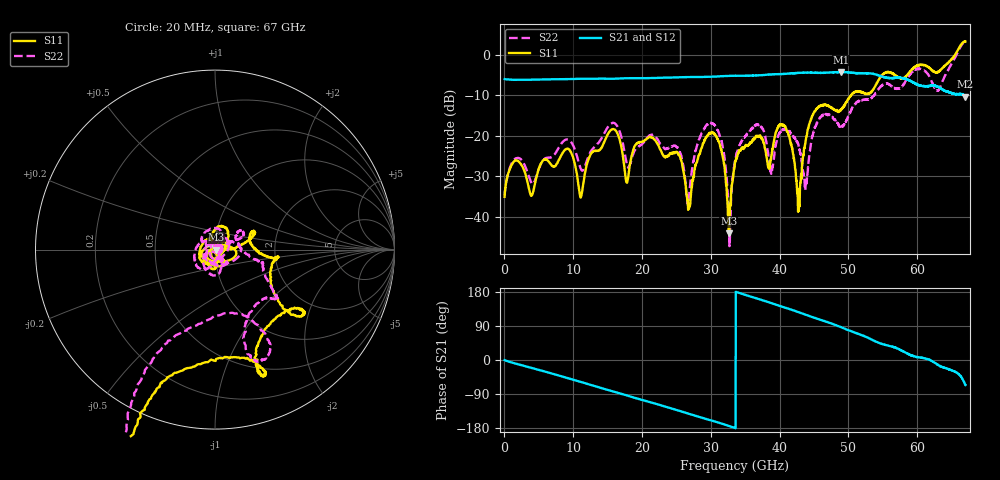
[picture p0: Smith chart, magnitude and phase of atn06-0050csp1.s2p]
!Keysight Technologies,N5247B,US58420632,A.14.00.23
!Date: Monday, April 25, 2022 11:31:55
!Correction: S11(C  2-Port  )
!S21(C  2-Port  )
!S12(C  2-Port  )
!S22(C  2-Port  )
!S2P File: Measurement: :
# Hz S  dB  R 50
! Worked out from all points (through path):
!   3350 points, 20 MHz to 67 GHz, reference 50 ohm
!   highest |S21| = -4.23 dB at 48.9 GHz (marker M1); lowest = -10.4 dB at 67 GHz (marker M2)
!   group delay of S21, straight-line fit = 16.5 ps
!   lowest |S11| = -44.1 dB at 32.6 GHz (marker M3), VSWR 1.01, Z = 50.6 - j0.0115 ohm
!   |S11| at or under -10 dB: start of sweep to 50.39 GHz
!   |S22| runs from -47.3 to 3.6 dB; largest |S21 - S12| = 0.0066
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2e7  -35.09 7.4  -5.99 -0.3  -5.99 -0.3  -34.72 6.2
9.1e9  -23.19 27.8  -6.00 -47.3  -6.00 -47.3  -20.91 36.7
1.12e10  -34.67 147.7  -5.90 -58.4  -5.91 -58.4  -28.47 130.2
1.554e10  -18.47 -17.6  -5.91 -81.6  -5.92 -81.6  -16.96 -9.7
1.778e10  -31.57 98.0  -5.78 -93.4  -5.78 -93.4  -26.99 84.1
2.236e10  -22.23 -50.6  -5.69 -117.5  -5.69 -117.5  -21.17 -44.9
2.536e10  -24.66 -67.1  -5.56 -133.8  -5.56 -133.8  -23.57 -49.9
2.668e10  -38.09 -101.3  -5.49 -141.2  -5.50 -141.2  -36.84 -109.2
3.042e10  -19.39 -89.9  -5.39 -161.4  -5.40 -161.4  -17.23 -83.7
3.178e10  -25.71 -78.5  -5.25 -169.0  -5.27 -169.1  -23.31 -61.6
3.26e10  -44.06 -1.0  -5.21 -173.8  -5.21 -173.9  -39.57 -18.0
3.352e10  -26.37 97.3  -5.18 -179.6  -5.17 -179.5  -26.20 129.7
3.688e10  -20.03 -138.1  -5.09 161.3  -5.07 161.4  -17.33 -132.4
3.88e10  -24.94 12.4  -4.86 149.8  -4.84 149.8  -29.19 -19.3
4.052e10  -17.30 73.5  -4.72 139.6  -4.73 139.6  -18.42 86.7
4.276e10  -38.41 55.7  -4.48 126.3  -4.45 126.3  -22.65 153.4
4.376e10  -21.63 1.2  -4.39 119.7  -4.41 119.9  -32.33 83.3
4.468e10  -15.34 13.0  -4.38 113.8  -4.41 113.8  -20.55 24.7
4.89e10  -13.61 6.0  -4.23 86.5  -4.27 86.7  -17.55 25.0
5.584e10  -4.26 -35.5  -5.72 37.6  -5.74 37.6  -7.20 -39.0
6.32e10  -3.99 -94.2  -8.08 -14.9  -8.03 -15.0  -8.34 -92.7
6.7e10  3.29 -108.3  -10.37 -66.2  -10.37 -66.3  3.55 -103.9
